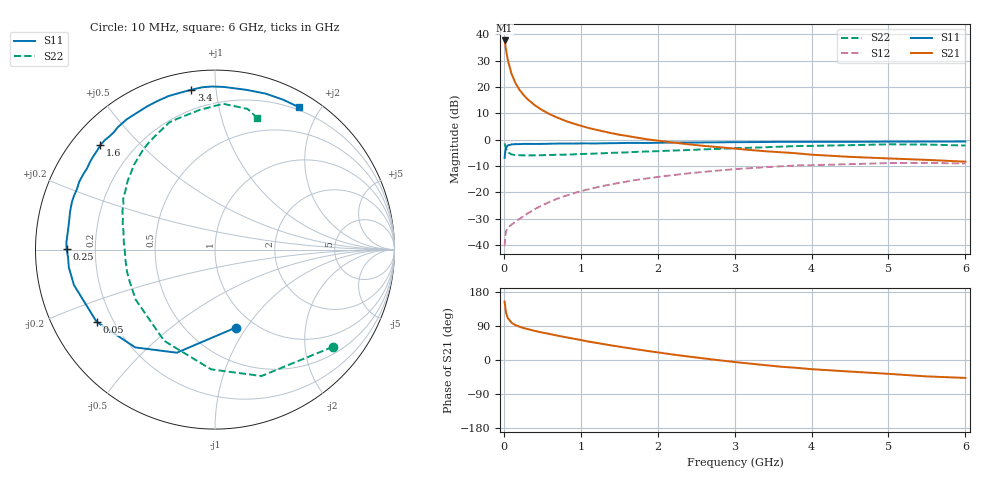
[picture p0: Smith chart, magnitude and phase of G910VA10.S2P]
! SIEMENS Small Signal Semiconductors
! BFG235
! Si NPN RF Bipolar Junction Transistor in SOT223
! VCE = 10 V  IC = 100 mA
! Common Emitter S-Parameters:  July  1994
# GHz  S  MA  R  50
!  f  S11  S21  S12  S22
! GHz  MAG  ANG  MAG  ANG  MAG  ANG  MAG  ANG
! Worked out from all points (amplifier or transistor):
!   40 points, 10 MHz to 6 GHz, reference 50 ohm
!   highest |S21| = 37.6 dB at 10 MHz (marker M1)
!   |S21| within 3 dB of that: start of sweep to 25.87 MHz
!   unconditionally stable (mu >= 1): 473.7 MHz to 1.429 GHz
!   at 200 MHz: K = 0.76, MSG = 24.6 dB, |S12| = -30.2 dB
!   at 1.5 GHz: K = 0.99, MSG = 9.1 dB, |S12| = -16.4 dB
!   at 6 GHz: K = 0.90, MSG = 0.4 dB, |S12| = -9.1 dB
!   S11 on the Smith chart (normalised r, x): 10 MHz: 0.82, -0.90; 50 MHz: 0.14, -0.28; 250 MHz: 0.09, +0.00; 1.6 GHz: 0.08, +0.39; 3.4 GHz: 0.09, +0.86; 6 GHz: 0.17, +1.73
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0.01  0.4494 -75.0  75.98 154.4  0.0095 65.6  0.8513 -39.5
0.02  0.6125 -110.3  61.23 136.2  0.0152 50.8  0.7505 -69.8
0.03  0.7032 -129.2  49.09 124.3  0.0184 42.9  0.6675 -91.9
0.05  0.7728 -148.6  33.19 111.2  0.0212 34.1  0.5818 -119.2
0.1  0.8103 -165.9  17.69 98.3  0.0244 35.3  0.5226 -147.8
0.15  0.8205 -173.1  11.92 92.1  0.0276 40.2  0.5074 -159.9
0.2  0.8198 -176.9  8.926 88.1  0.031 44.0  0.5052 -166.4
0.25  0.827 179.6  7.185 84.7  0.0348 48.5  0.502 -170.7
0.3  0.8289 177.2  6.002 82.1  0.0388 51.7  0.5026 -174.1
0.4  0.8259 172.4  4.512 76.9  0.0477 55.5  0.5022 -178.7
0.5  0.8286 168.6  3.606 72.4  0.0567 57.5  0.506 177.8
0.6  0.8346 165.4  3.009 68.5  0.0662 58.2  0.5104 174.6
0.8  0.841 159.1  2.268 60.3  0.0855 58.3  0.518 169.5
1.1  0.8455 149.8  1.663 48.6  0.1141 55.4  0.5379 162.9
1.4  0.8542 142.7  1.324 38.4  0.1417 51.2  0.5596 157.0
1.6  0.8639 137.6  1.174 32.1  0.1601 47.9  0.5719 153.1
2.2  0.877 124.1  0.878 14.4  0.2118 37.5  0.6204 141.5
3.2  0.8951 102.7  0.635 -9.5  0.2871 18.2  0.6992 122.2
3.4  0.9002 98.4  0.601 -13.7  0.2991 14.1  0.7154 117.8
4.5  0.9071 78.8  0.47 -30.5  0.3418 -7.1  0.7832 96.2
5.5  0.9172 65.6  0.412 -43.3  0.362 -25.7  0.8048 77.0
6  0.9211 59.6  0.381 -47.3  0.3512 -32.4  0.7709 72.3
